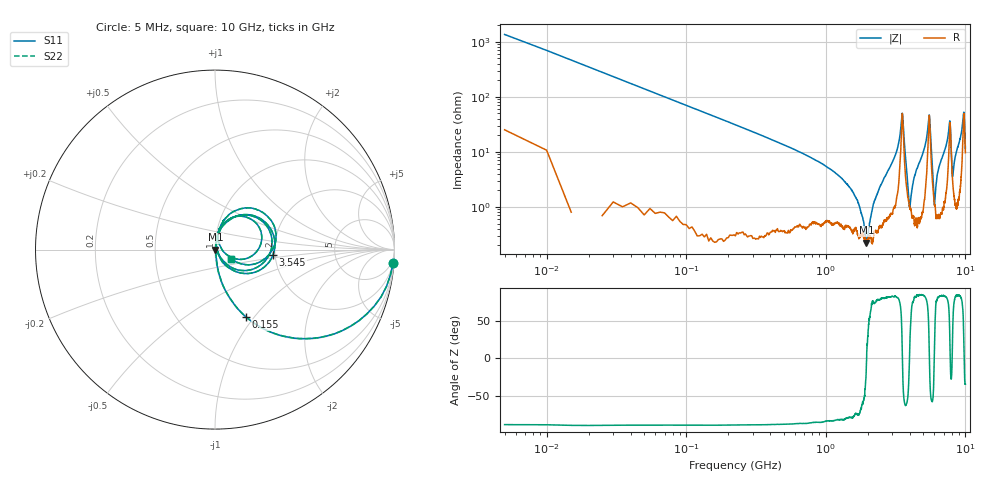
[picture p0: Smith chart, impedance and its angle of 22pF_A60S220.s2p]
! Amotech Co.,Ltd.
! http://www.amotech.co.kr/
! Part Number: A60S220
! These Parameters are Measured in Series Mode Connection
! Operation Temp=25[degC], DC Bias Voltage=0[V]
! Freq. Start=5[MHz] Stop=10[GHz], 2000[Steps]
! Date: Monday, July 13, 2020, 01:38:32
# GHZ S RI R 50.000000
!Freq.(Hz) S11(Real) S11(Imag) S21(Real) S21(Imag) S12(Real) S12(Imag) S22(Real) S22(Imag)
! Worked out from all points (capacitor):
!   2000 points, 5 MHz to 10 GHz, reference 50 ohm
!   read as one part in series: C = 22.5 pF near 55 MHz
!   lowest |Z| = 224 mohm at 1.955 GHz (marker M1)
!   series resonance near 1.961 GHz, so ESL is about 290 pH
!   S11 on the Smith chart (normalised r, x): 5 MHz: 2, -27; 155 MHz: 1.00, -0.91; 3.545 GHz: 1.95, -0.13; 10 GHz: 1.19, -0.13
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0.005  0.9933 -0.0728  0.00669 0.0728  0.00669 0.0728  0.9933 -0.0728
0.07  0.5032 -0.4961  0.4968 0.4961  0.4968 0.4961  0.5032 -0.4961
0.155  0.1725 -0.3752  0.8275 0.3752  0.8275 0.3752  0.1725 -0.3752
0.555  0.0174 -0.1173  0.9826 0.1173  0.9826 0.1173  0.0174 -0.1173
1.675  0.00385 -0.0129  0.9961 0.0129  0.9961 0.0129  0.00385 -0.0129
1.955  0.00222 -0.000226  0.9978 0.000226  0.9978 0.000226  0.00222 -0.000226
2.265  0.00387 0.0133  0.9961 -0.0133  0.9961 -0.0133  0.00387 0.0133
3.34  0.0484 0.1372  0.9516 -0.1372  0.9516 -0.1372  0.0484 0.1372
3.545  0.3229 -0.0306  0.6771 0.0306  0.6771 0.0306  0.3229 -0.0306
3.99  0.00964 0.00171  0.9904 -0.00171  0.9904 -0.00171  0.00964 0.00171
4.3  0.00639 0.0341  0.9936 -0.0341  0.9936 -0.0341  0.00639 0.0341
5.005  0.0191 0.0983  0.9809 -0.0983  0.9809 -0.0983  0.0191 0.0983
5.52  0.3146 0.00654  0.6854 -0.00654  0.6854 -0.00654  0.3146 0.00654
6.005  0.0107 0.00191  0.9893 -0.00191  0.9893 -0.00191  0.0107 0.00191
6.29  0.0083 0.038  0.9917 -0.038  0.9917 -0.038  0.0083 0.038
6.67  0.0121 0.066  0.9879 -0.066  0.9879 -0.066  0.0121 0.066
7.715  0.2431 0.1289  0.7569 -0.1289  0.7569 -0.1289  0.2431 0.1289
8.065  0.0343 0.00865  0.9657 -0.00865  0.9657 -0.00865  0.0343 0.00865
8.335  0.0178 0.0623  0.9822 -0.0623  0.9822 -0.0623  0.0178 0.0623
9.34  0.0745 0.1909  0.9255 -0.1909  0.9255 -0.1909  0.0745 0.1909
9.7  0.3146 0.1597  0.6854 -0.1597  0.6854 -0.1597  0.3146 0.1597
10  0.0914 -0.055  0.9086 0.055  0.9086 0.055  0.0914 -0.055
